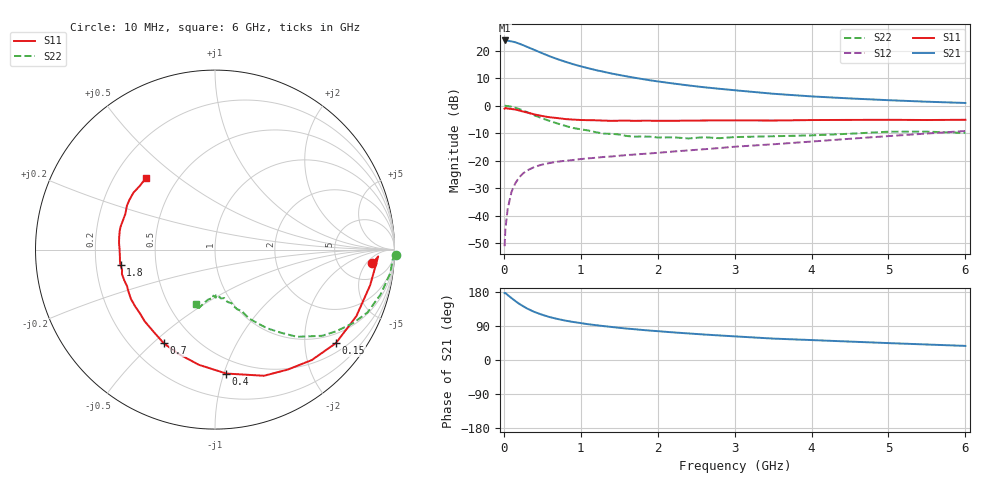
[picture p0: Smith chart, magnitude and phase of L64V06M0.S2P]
!  INFINEON TECHNOLOGIES Small Signal Semiconductors
! BFR380L3 , Si-NPN RF-Transistor in TSLP-3-1
!  Vce=4 V,  Ic=6 mA
! Common Emitter S-Parameters:  07. March 2005
#  GHz  S  MA  R  50
! f  S11  S21  S12  S22
! GHz  Mag  Ang  Mag  Ang  Mag  Ang  Mag  Ang
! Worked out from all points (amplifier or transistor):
!   36 points, 10 MHz to 6 GHz, reference 50 ohm
!   highest |S21| = 23.7 dB at 10 MHz (marker M1)
!   |S21| within 3 dB of that: start of sweep to 359.5 MHz
!   unconditionally stable (mu >= 1): 2.56 GHz to 4.655 GHz
!   at 250 MHz: K = 0.18, MSG = 23.3 dB, |S12| = -24.6 dB
!   at 1.4 GHz: K = 0.77, MSG = 15.1 dB, |S12| = -18.5 dB
!   at 6 GHz: K = 0.94, MSG = 5.1 dB, |S12| = -9.2 dB
!   S11 on the Smith chart (normalised r, x): 10 MHz: 11, -7; 150 MHz: 0.73, -2.76; 400 MHz: 0.38, -1.02; 700 MHz: 0.34, -0.54; 1.8 GHz: 0.31, -0.07; 6 GHz: 0.33, +0.39
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0.01  0.8805 -5.0  15.33 176.5  0.0028 80.8  1.011 -1.6
0.02  0.91 -2.4  15.21 176.8  0.0057 94.2  0.9912 -3.2
0.05  0.8868 -13.0  15.18 171.4  0.0133 86.0  0.9854 -7.7
0.1  0.8705 -25.2  14.73 163.4  0.0273 77.2  0.9557 -15.2
0.15  0.8518 -37.7  14.19 155.5  0.0391 71.0  0.9188 -22.4
0.2  0.8182 -48.8  13.42 148.2  0.0501 66.7  0.8712 -28.1
0.25  0.782 -58.7  12.6 142.1  0.0587 61.3  0.8147 -33.9
0.3  0.7539 -68.8  11.76 136.1  0.0662 58.1  0.7664 -38.8
0.4  0.6934 -84.8  10.28 126.6  0.0774 51.8  0.6667 -46.8
0.5  0.6483 -97.9  8.973 119.3  0.0853 48.4  0.5881 -51.8
0.6  0.6152 -109.6  7.864 113.0  0.091 45.6  0.5253 -56.5
0.7  0.5951 -118.6  6.998 108.2  0.0961 44.5  0.4737 -60.0
0.9  0.5594 -134.5  5.68 100.4  0.103 43.0  0.3929 -65.5
1.1  0.5458 -144.8  4.781 94.3  0.1104 43.5  0.3539 -69.7
1.4  0.5305 -157.5  3.842 87.2  0.1195 44.7  0.3084 -74.1
1.8  0.5335 -170.6  3.054 79.3  0.1328 47.6  0.2748 -80.2
2.2  0.5314 -179.7  2.534 72.9  0.1469 50.4  0.2664 -84.7
2.8  0.5411 168.7  2.03 64.8  0.1698 54.4  0.2569 -92.1
3.5  0.5375 158.3  1.649 56.5  0.199 56.7  0.2784 -97.1
4.5  0.5516 149.7  1.355 48.6  0.2507 60.1  0.3095 -102.3
5.5  0.5492 139.9  1.182 40.9  0.3121 60.2  0.3377 -107.0
6  0.5546 133.6  1.121 37.2  0.347 59.1  0.3199 -109.2
